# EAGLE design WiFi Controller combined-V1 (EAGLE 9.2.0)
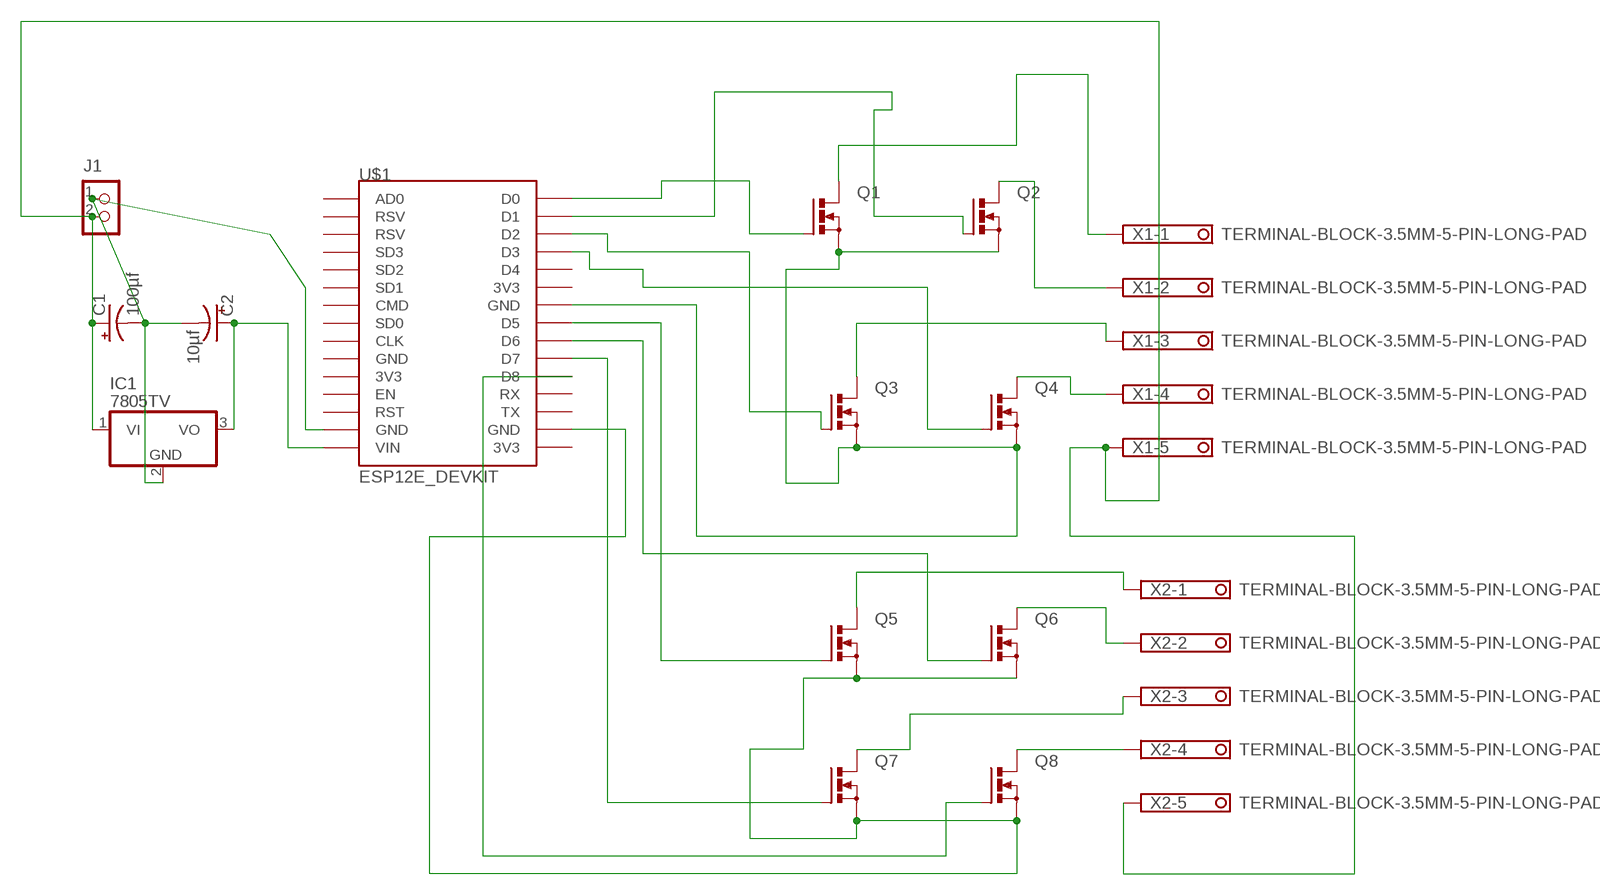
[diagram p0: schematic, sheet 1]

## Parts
C1  100µf  CPOL-USE1.8-4  [E1,8-4]
C2  10µf  CPOL-USE1.8-4  [E1,8-4]
IC1  7805TV  [TO220V]
J1  CON_TERMINAL_BLOCK_02-5MM  [TERMINAL_BLOCK_2P_5]
Q1  PMOSFET_NTO220BV  [TO220BV]
Q2  PMOSFET_NTO220BV  [TO220BV]
Q3  PMOSFET_NTO220BV  [TO220BV]
Q4  PMOSFET_NTO220BV  [TO220BV]
Q5  PMOSFET_NTO220BV  [TO220BV]
Q6  PMOSFET_NTO220BV  [TO220BV]
Q7  PMOSFET_NTO220BV  [TO220BV]
Q8  PMOSFET_NTO220BV  [TO220BV]
U$1  ESP12E_DEVKIT  [ESP12E_DEVKIT]
X1  TERMINAL-BLOCK-3.5MM-5-PIN-LONG-PAD  [TERMINAL-BLOCK-5-PIN-3.5MM-LONG-PAD]
X2  TERMINAL-BLOCK-3.5MM-5-PIN-LONG-PAD  [TERMINAL-BLOCK-5-PIN-3.5MM-LONG-PAD]

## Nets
N$1: C1.+ IC1.1(VI) J1.2 X1.5 X2.5
N$2: C1.- C2.- IC1.2(GND) J1.1 U$1.GND@1(GND)
N$3: C2.+ IC1.3(VO) U$1.VIN
N$4: Q1.G U$1.D0
N$5: Q2.G U$1.D1
N$6: Q3.G U$1.D2
N$7: Q4.G U$1.D3
N$8: Q1.S Q2.S Q3.S Q4.S U$1.GND@2(GND)
N$9: Q5.D X2.1
N$10: Q6.D X2.2
N$11: Q7.D X2.3
N$12: Q8.D X2.4
N$13: Q5.S Q6.S Q7.S Q8.S U$1.GND@3(GND)
N$14: Q1.D X1.1
N$15: Q3.D X1.3
N$16: Q2.D X1.2
N$17: Q4.D X1.4
N$18: Q5.G U$1.D5
N$19: Q6.G U$1.D6
N$20: Q7.G U$1.D7
N$21: Q8.G U$1.D8
Unconnected: U$1.3V3@0(3V3) U$1.3V3@1(3V3) U$1.3V3@2(3V3) U$1.AD0 U$1.CLK U$1.CMD U$1.D4 U$1.EN U$1.GND@0(GND) U$1.RST U$1.RSV@0(RSV) U$1.RSV@1(RSV) U$1.RX U$1.SD0 U$1.SD1 U$1.SD2 U$1.SD3 U$1.TX

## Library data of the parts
C1 C2 = rcl:CPOL-US: POLARIZED CAPACITOR, American symbol; SPICEPREFIX: C
IC1 = linear:78*: Positive VOLTAGE REGULATOR Source: http://cache.national.com/ds/LM/LM78L05.pdf http://www.fairchildsemi.com/ds/LM/LM7805.pdf
J1 = dp_devices:CON_TERMINAL_BLOCK_02: 2 poles wire to board terminal block
Q1-Q8 = transistor-power:PMOSFET_N: Power MOSFET N-Channel
U$1 = ESP12E_DEVKIT:ESP12E_DEVKIT: ESP12E DEVKIT BOARD
X1 X2 = Rembrandt Electronics - Terminal Block 3-5mm v1-0:TERMINAL-BLOCK-3.5MM-5-PIN: Terminal Block 3.5mm Pitch: 3,5 mm Number of pins: 5 Created by Rembrandt Electronics www.rembrandtelectronics.com

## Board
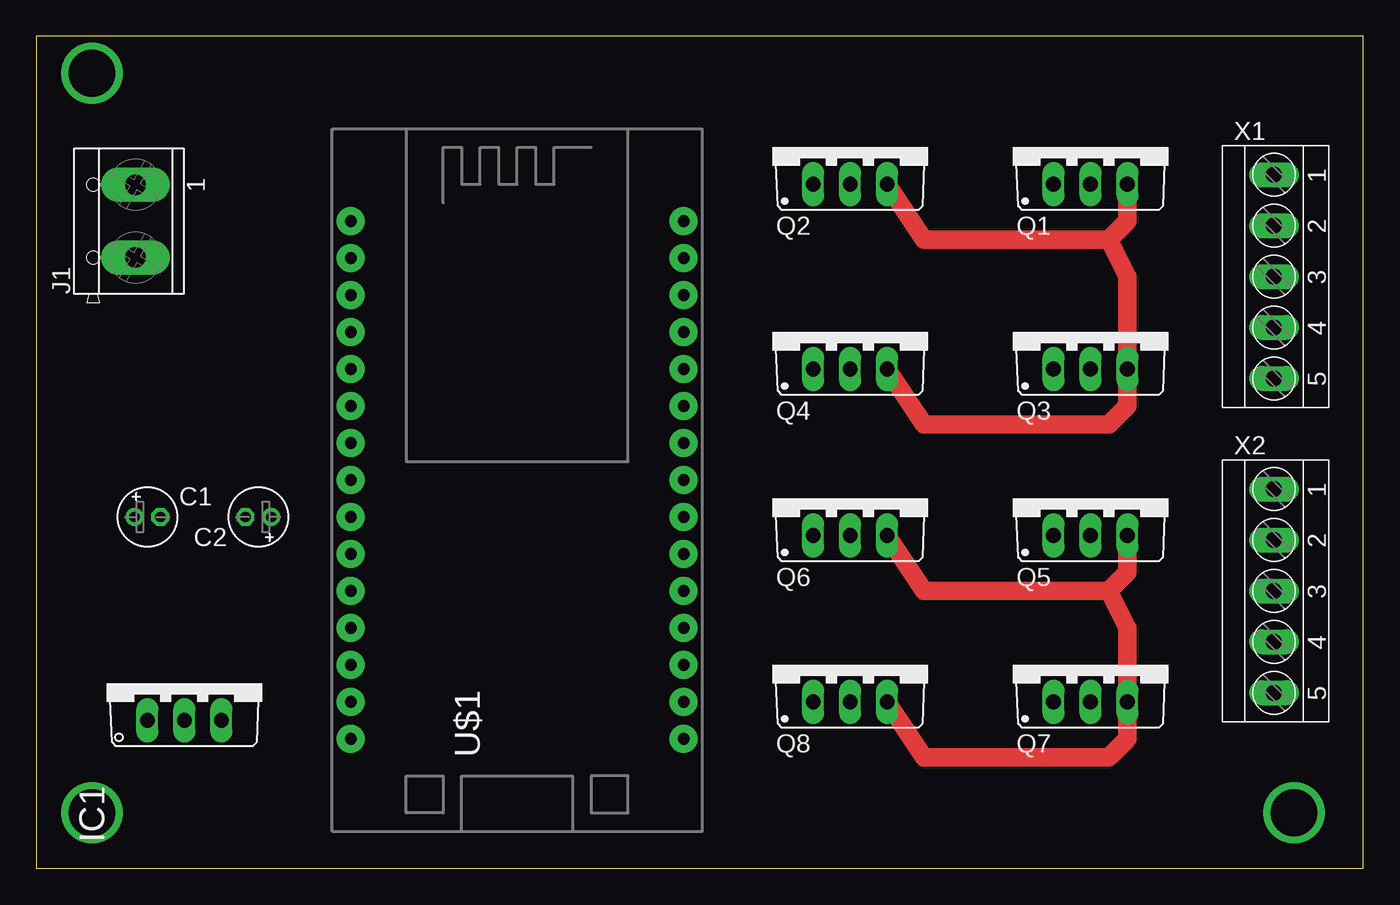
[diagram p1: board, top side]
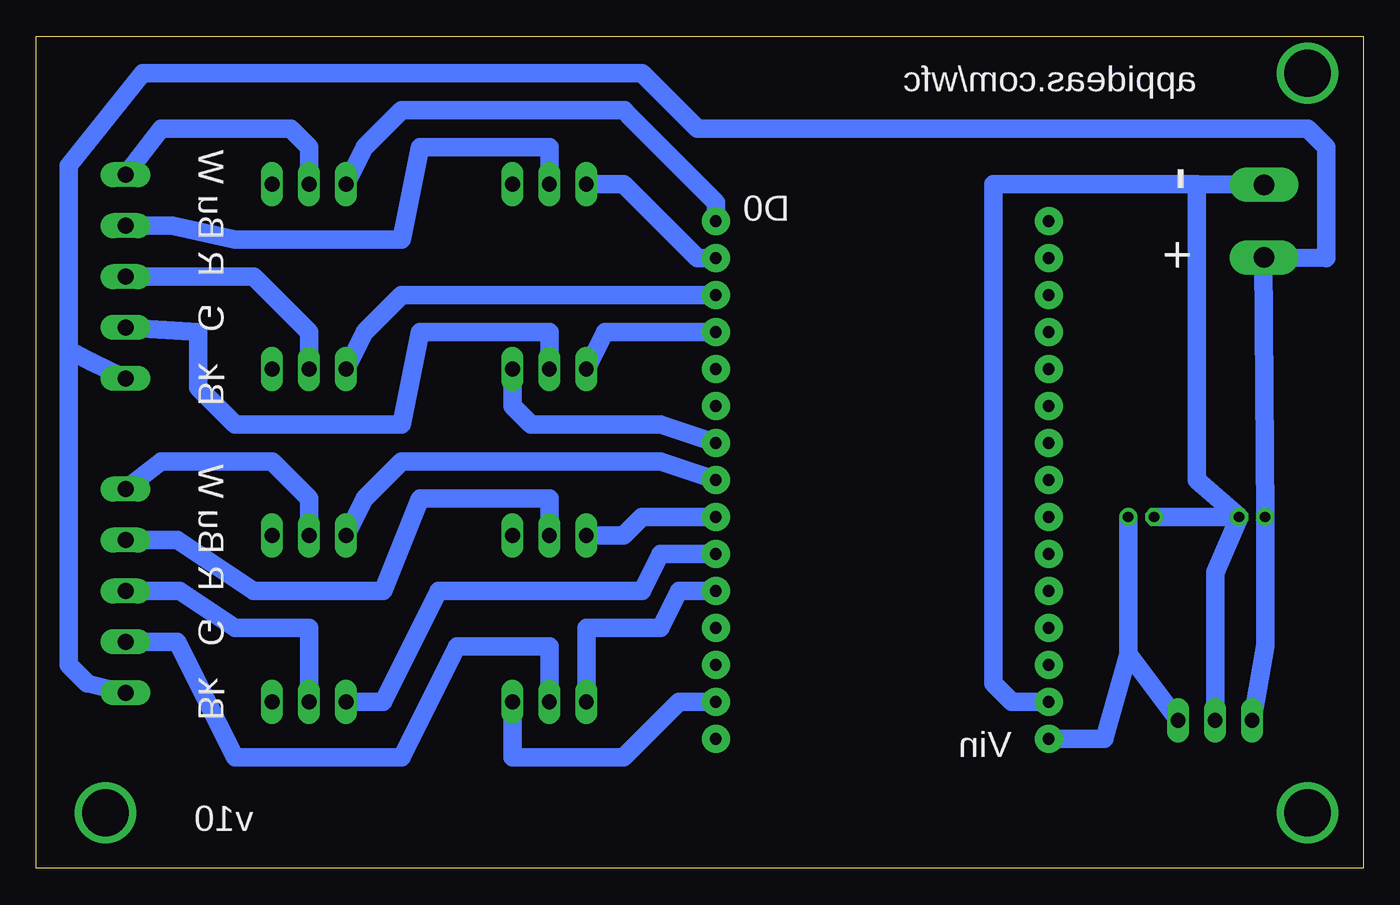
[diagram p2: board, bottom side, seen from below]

Size 91.11 x 57.14 mm. Coordinates in mm from the lower left corner, seen from the top.
Outline: 0,0 91.11,0 91.11,57.14 0,57.14 0,0
Copper layers (1*16): Top 0.035mm / dielectric 1.5mm / Bottom 0.035mm
Design rules "default": minimum track width 6mil, minimum drill 0.35mm, track to track 6mil, track to pad 6mil, pad to pad 6mil, via to via 6mil, smd to smd 6mil, copper to edge 40mil, drill to drill 6mil, minimum pad ring 10mil, minimum via ring 8mil, stop-mask expansion 4mil, vias tented up to drill 0mil, thermal gap 10mil

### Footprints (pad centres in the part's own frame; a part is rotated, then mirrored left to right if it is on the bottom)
E1,8-4 = drill 0.711 pad 1.168: + -0.889,0 | drill 0.711 pad 1.168 octagon: - 0.889,0
TO220V = drill 1.016 long: 1 -2.54,-2.54; 2 0,-2.54; 3 2.54,-2.54
TERMINAL_BLOCK_2P_5 = drill 1.4 pad 2.38 long: 1 2.5,-0.45; 2 -2.5,-0.45
TO220BV = drill 1.016 long: D 0,-2.54; G -2.54,-2.54; S 2.54,-2.54
ESP12E_DEVKIT = drill 0.8 pad 1.93: 3V3@0 -11.43,-7.62; 3V3@1 11.43,5.08; 3V3@2 11.43,-17.78; AD0 -11.43,17.78; CLK -11.43,-2.54; CMD -11.43,2.54; D0 11.43,17.78; D1 11.43,15.24; D2 11.43,12.7; D3 11.43,10.16; D4 11.43,7.62; D5 11.43,0; D6 11.43,-2.54; D7 11.43,-5.08; D8 11.43,-7.62; EN -11.43,-10.16; GND@0 -11.43,-5.08; GND@1 -11.43,-15.24; GND@2 11.43,2.54; GND@3 11.43,-15.24; RST -11.43,-12.7; RSV@0 -11.43,15.24; RSV@1 -11.43,12.7; RX 11.43,-10.16; SD0 -11.43,0; SD1 -11.43,5.08; SD2 -11.43,7.62; SD3 -11.43,10.16; TX 11.43,-12.7; VIN -11.43,-17.78
TERMINAL-BLOCK-5-PIN-3.5MM-LONG-PAD = drill 1.1 pad 1.7 long: 1 -7,-0.1; 2 -3.5,-0.1; 3 0,-0.1; 4 3.5,-0.1; 5 7,-0.1

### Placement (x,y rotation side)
C1  7.62,24.13 0 top
C2  15.24,24.13 180 top
IC1  10.16,12.7 0 top
J1  6.35,44.45 90 top
Q1  72.39,49.53 0 top
Q2  55.88,49.53 0 top
Q3  72.39,36.83 0 top
Q4  55.88,36.83 0 top
Q5  72.39,25.4 0 top
Q6  55.88,25.4 0 top
Q7  72.39,13.97 0 top
Q8  55.88,13.97 0 top
U$1  33.02,26.67 0 top
X1  85.09,40.64 270 top
X2  85.09,19.05 270 top

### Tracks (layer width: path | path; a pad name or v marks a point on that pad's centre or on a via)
N$1
  Bottom 1.27: IC1.1 6.73,15.28 C1.+ 6.84,41.91 J1.2 2.54,41.91 2.54,49.53 3.81,50.8 45.72,50.8 49.53,54.61 83.82,54.61 88.9,48.26 88.9,35.56 | 88.9,35.56 88.39,35.31 87.37,34.81 X1.5 | X2.5 87.63,12.7 88.9,13.97 88.9,35.56
N$2
  Bottom 1.27: C1.- C2.- | 11.43,46.99 25.4,46.99 25.4,12.7 24.13,11.43 U$1.GND@1 | C1.- 10.16,20.32 IC1.2 | J1.1 11.43,46.99 | C1.- 11.43,26.67 11.43,46.99
N$3
  Bottom 1.27: 16.13,14.73 C2.+ | IC1.3 16.13,14.73 | U$1.VIN 17.78,8.89 16.13,14.73
N$4
  Bottom 1.27: Q1.G 68.58,49.53 66.04,52.07 50.72,52.07 50.48,51.75 44.45,45.72 U$1.D0
N$5
  Bottom 1.27: Q2.G 50.8,46.99 45.72,41.91 U$1.D1
N$6
  Bottom 1.27: Q3.G 68.58,36.83 66.04,39.37 U$1.D2
N$7
  Bottom 1.27: Q4.G 52.07,36.83 U$1.D3
N$8
  Top 1.27: Q1.S 74.93,44.45 73.66,43.18 | 73.66,43.18 60.96,43.18 Q2.S | Q4.S 60.96,30.48 73.66,30.48 74.93,31.75 Q3.S 74.93,40.64 73.66,43.18
  Bottom 1.27: Q4.S 58.42,31.75 57.15,30.48 48.26,30.48 U$1.GND@2
N$9
  Bottom 1.27: Q5.D 72.39,25.4 74.93,27.94 82.55,27.94 X2.1
N$10
  Bottom 1.27: Q6.D 55.88,25.4 64.77,25.4 67.31,19.05 76.2,19.05 81.45,22.55 X2.2
N$11
  Bottom 1.27: X2.3 81.28,19.05 77.47,16.51 72.39,16.51 Q7.D
N$12
  Bottom 1.27: Q8.D 55.88,15.24 62.23,15.24 66.04,7.62 77.47,7.62 81.44,15.55 X2.4
N$13
  Top 1.27: Q5.S 74.93,20.32 73.66,19.05 | 73.66,19.05 60.96,19.05 Q6.S | Q8.S 60.96,7.62 73.66,7.62 74.93,8.89 Q7.S 74.93,16.51 73.66,19.05
  Bottom 1.27: U$1.GND@3 46.99,11.43 50.8,7.62 58.42,7.62 Q8.S
N$14
  Bottom 1.27: Q1.D 72.39,49.53 73.66,50.8 82.55,50.8 X1.1
N$15
  Bottom 1.27: Q3.D 72.39,36.83 76.2,40.64 X1.3
N$16
  Bottom 1.27: Q2.D 55.88,49.53 64.77,49.53 66.04,43.18 77.47,43.18 81.8,44.14 X1.2
N$17
  Bottom 1.27: Q4.D 55.88,36.83 64.77,36.83 66.04,30.48 77.47,30.48 80.01,33.02 80.01,36.83 X1.4
N$18
  Bottom 1.27: Q5.G 68.58,25.4 66.04,27.94 48.26,27.94 U$1.D5
N$19
  Bottom 1.27: Q6.G 50.8,22.86 49.53,24.13 U$1.D6
N$20
  Bottom 1.27: Q7.G 67.31,11.43 63.5,19.05 49.53,19.05 48.26,21.59 U$1.D7
N$21
  Bottom 1.27: Q8.G 53.34,16.51 48.26,16.51 46.99,19.05 U$1.D8
N$22  (via drill 3.2)
  other vias: 3.81,54.61
N$23  (via drill 3.2)
  other vias: 3.81,3.81
N$24  (via drill 3.2)
  other vias: 86.36,3.81

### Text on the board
bPlace: appideas.com/wfc | - | W | D0 | + | Bu | R | G | Bk | W | Bu | R | G | Bk | Vin | v10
